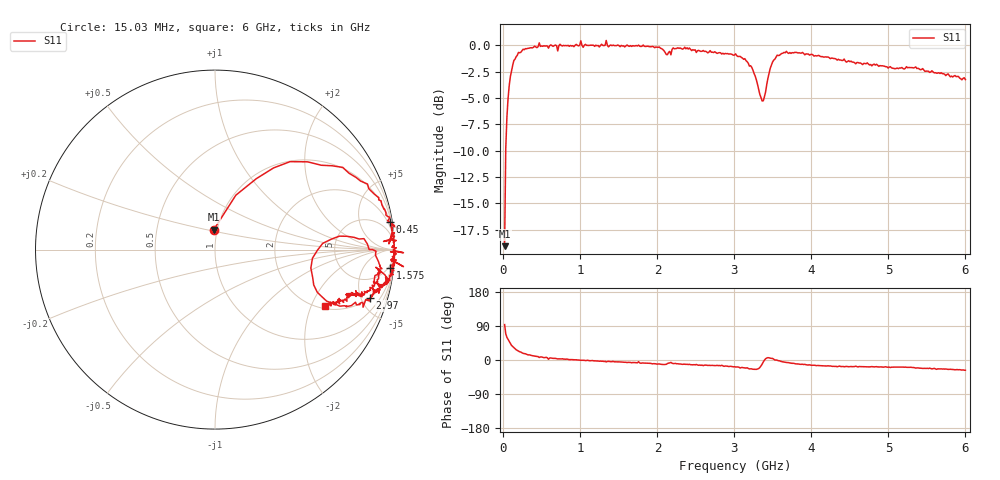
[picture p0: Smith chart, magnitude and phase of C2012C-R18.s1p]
!	Network	Analyzer	HP8753E.07.74:	Oct	30	2002	Serial	No.	JP38451487
!	Hewlett-Packard
!	7	Sep	2009	12:16:19
!	Frequency	S11
#	HZ	S	RI	R	50
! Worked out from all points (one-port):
!   400 points, 15.03 MHz to 6 GHz, reference 50 ohm
!   lowest |S11| = -19.1 dB at 15.03 MHz (marker M1), VSWR 1.25, Z = 48.1 + j10.8 ohm
!   |S11| at or under -10 dB: start of sweep to 29.67 MHz
!   S11 on the Smith chart (normalised r, x): 15.03 MHz: 0.96, +0.22; 450 MHz: 1, +13; 1.575 GHz: 3, -18; 2.97 GHz: 1.99, -5.92; 6 GHz: 2.12, -2.52
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1.502992e7  -0.00665 0.111
3.002985e7  0.116 0.303
6.00297e7  0.326 0.455
9.002955e7  0.516 0.489
1.95029e8  0.85 0.365
4.500278e8  0.973 0.154
5.550272e8  0.986 0.124
5.850271e8  0.969 0.0319
7.650262e8  0.991 0.058
1.005025e9  1.05 -0.0174
1.245024e9  0.98 -0.0559
1.335023e9  1.05 -0.095
1.515022e9  0.981 -0.0872
1.575022e9  0.977 -0.103
2.02502e9  0.965 -0.178
2.115019e9  0.886 -0.179
2.175019e9  0.896 -0.0985
2.265019e9  0.959 -0.167
2.970015e9  0.864 -0.269
3.015015e9  0.864 -0.287
3.240014e9  0.695 -0.315
3.360013e9  0.534 -0.103
3.450013e9  0.734 0.0742
3.555012e9  0.897 -0.00885
3.765011e9  0.91 -0.138
4.515007e9  0.803 -0.249
5.265004e9  0.74 -0.26
6e9  0.612 -0.313
